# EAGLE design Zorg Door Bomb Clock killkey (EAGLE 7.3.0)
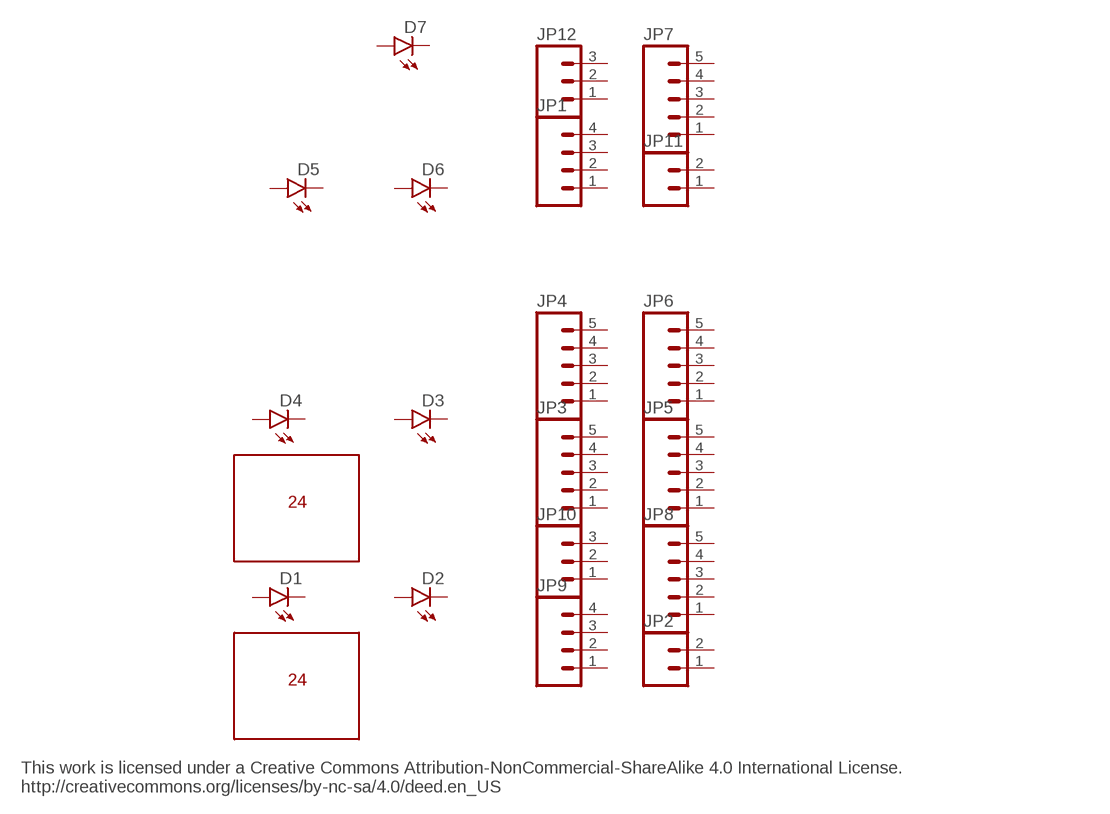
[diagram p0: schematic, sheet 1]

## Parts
D1  LED1206  [LED-1206]
D2  LED1206  [LED-1206]
D3  LED1206  [LED-1206]
D4  LED1206  [LED-1206]
D5  LED1206  [LED-1206]
D6  LED1206  [LED-1206]
D7  LED1206  [LED-1206]
JP1  M041X04_NO_SILK  [1X04_NO_SILK]
JP2  M021X02_NO_SILK  [1X02_NO_SILK]
JP3  M05NO_SILK  [1X05_NO_SILK]
JP4  M05NO_SILK  [1X05_NO_SILK]
JP5  M05NO_SILK  [1X05_NO_SILK]
JP6  M05NO_SILK  [1X05_NO_SILK]
JP7  M05NO_SILK  [1X05_NO_SILK]
JP8  M05NO_SILK  [1X05_NO_SILK]
JP9  M041X04_NO_SILK  [1X04_NO_SILK]
JP10  M031X03_NO_SILK  [1X03_NO_SILK]
JP11  M021X02_NO_SILK  [1X02_NO_SILK]
JP12  M031X03_NO_SILK  [1X03_NO_SILK]
U$1  SOIC24  [SOIC24]
U$2  SOIC24  [SOIC24]
Unconnected: D1.A D1.C D2.A D2.C D3.A D3.C D4.A D4.C D5.A D5.C D6.A D6.C D7.A D7.C JP1.1 JP1.2 JP1.3 JP1.4 JP2.1 JP2.2 JP3.1 JP3.2 JP3.3 JP3.4 JP3.5 JP4.1 JP4.2 JP4.3 JP4.4 JP4.5 JP5.1 JP5.2 JP5.3 JP5.4 JP5.5 JP6.1 JP6.2 JP6.3 JP6.4 JP6.5 JP7.1 JP7.2 JP7.3 JP7.4 JP7.5 JP8.1 JP8.2 JP8.3 JP8.4 JP8.5 JP9.1 JP9.2 JP9.3 JP9.4 JP10.1 JP10.2 JP10.3 JP11.1 JP11.2 JP12.1 JP12.2 JP12.3

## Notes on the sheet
- This work is licensed under a Creative Commons Attribution-NonCommercial-ShareAlike 4.0 International License.
  http://creativecommons.org/licenses/by-nc-sa/4.0/deed.en_US

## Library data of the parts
D1-D7 = SparkFun-LED:LED: LEDs
JP1 JP9 = zorg header 1:M04: Header 4 Standard 4-pin 0.1" header. Use with straight break away headers (SKU : PRT-00116), right angle break away headers (PRT-00553), swiss pins (PRT-00743), machine pins (PRT-00117), and female headers (PRT-00115). Molex polarized connector foot print use with SKU : PRT-08231 with associated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; PROD_ID: CONN-09696
JP2 JP11 = zorg header 1:M02: Standard 2-pin 0.1" header. Use with
JP3-JP8 = zorg header 1:M05: Header 5 Standard 5-pin 0.1" header. Use with straight break away headers (SKU : PRT-00116), right angle break away headers (PRT-00553), swiss pins (PRT-00743), machine pins (PRT-00117), and female headers (PRT-00115). Molex polarized connector foot print use with SKU : PRT-08230 with associated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
JP10 JP12 = zorg header 1:M03: Header 3 Standard 3-pin 0.1" header. Use with straight break away headers (SKU : PRT-00116), right angle break away headers (PRT-00553), swiss pins (PRT-00743), machine pins (PRT-00117), and female headers (PRT-00115). Molex polarized connector foot print use with SKU : PRT-08232 with associated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
U$1 U$2 = soic24:SOIC24

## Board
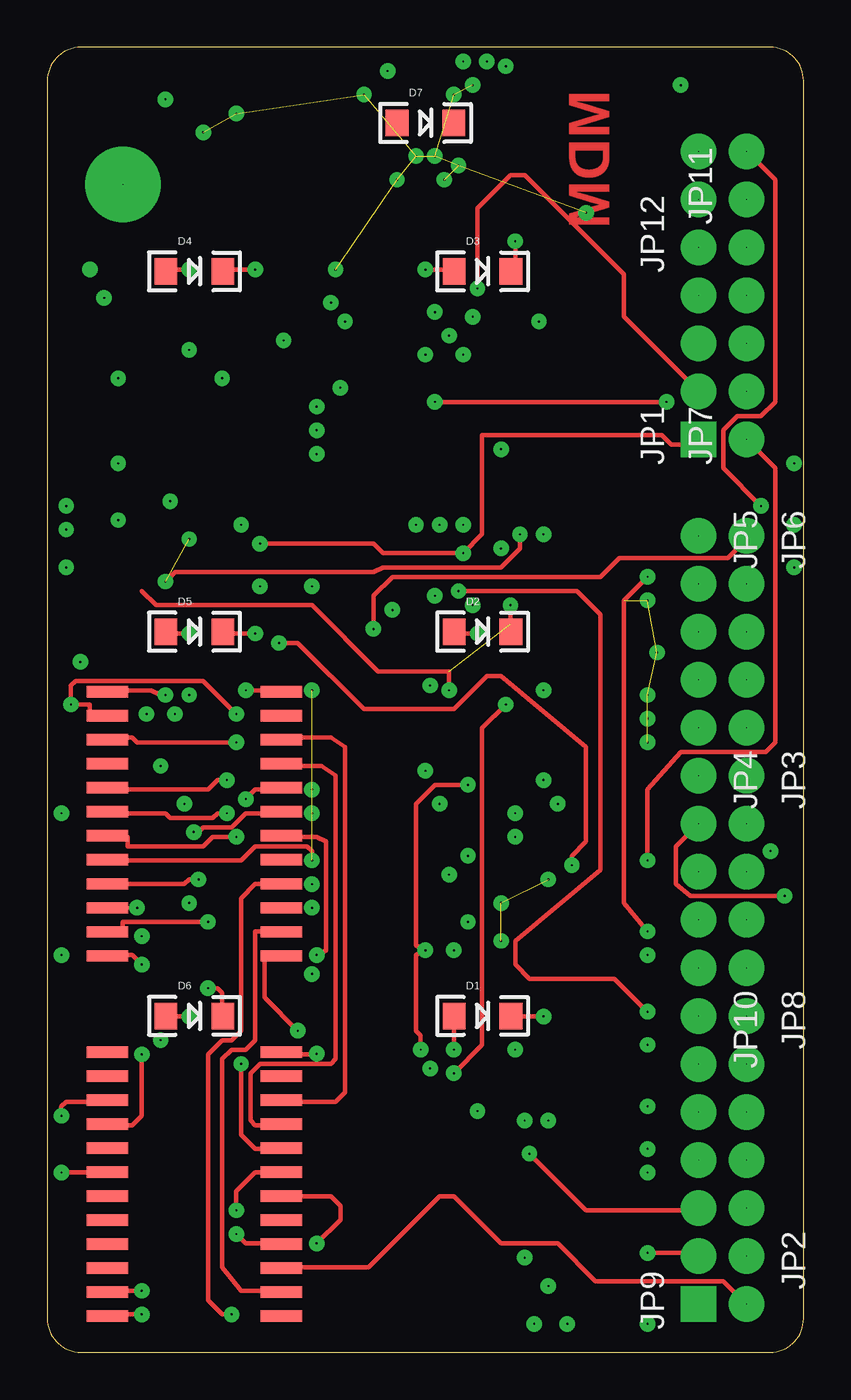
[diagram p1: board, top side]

Size 40 x 69 mm. Coordinates in mm from the lower left corner, seen from the top.
Outline: 0,67.23 0,1.77 arc90 1.77,0 38.23,0 arc90 40,1.77 40,67.23 arc90 38.23,69 1.77,69 arc90 0,67.23
Copper layers (1*16): Top 0.035mm / dielectric 1.5mm / Bottom 0.035mm
Design rules "default": minimum track width 10mil, minimum drill 24mil, track to track 8mil, track to pad 8mil, pad to pad 8mil, via to via 8mil, smd to smd 8mil, copper to edge 40mil, drill to drill 8mil, minimum pad ring 10mil, minimum via ring 8mil, stop-mask expansion 4mil, vias tented up to drill 0mil, thermal gap 10mil

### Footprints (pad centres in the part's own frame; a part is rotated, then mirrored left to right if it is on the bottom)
LED-1206 = smd 1.2 x 1.4: A -1.5,0; C 1.5,0
1X04_NO_SILK = drill 0.003 pad 1.88 square: 1 0,0 | drill 0.003 pad 1.88: 2 2.54,0; 3 5.08,0; 4 7.62,0
1X02_NO_SILK = drill 0.025 pad 1.88: 1 0,0; 2 2.54,0
1X05_NO_SILK = drill 0.025 pad 1.88: 1 0,0; 2 2.54,0; 3 5.08,0; 4 7.62,0; 5 10.16,0
1X03_NO_SILK = drill 0.025 pad 1.88: 1 0,0; 2 2.54,0; 3 5.08,0
SOIC24 = smd 2.2 x 0.6: 1 10.95,0.635; 2 10.95,1.905; 3 10.95,3.175; 4 10.95,4.445; 5 10.95,5.715; 6 10.95,6.985; 7 10.95,8.255; 8 10.95,9.525; 9 1.75,9.525; 10 1.75,8.255; 11 1.75,6.985; 12 1.75,5.715; 13 1.75,4.445; 14 1.75,3.175; 15 1.75,1.905; 16 1.75,0.635; 17 10.95,12.065; 18 1.75,14.605; 19 10.95,10.795; 20 10.95,13.335; 21 10.95,14.605; 22 1.75,13.335; 31 1.75,12.065; 32 1.75,10.795

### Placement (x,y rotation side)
D1  23.02,17.78 0 top
D2  23.02,38.1 0 top
D3  23.02,57.15 0 top
D4  7.78,57.15 0 top
D5  7.78,38.1 0 top
D6  7.78,17.78 0 top
D7  20,65 0 top
JP1  34.45,48.26 90 top
JP2  36.99,5.08 270 top
JP3  36.99,30.48 270 top
JP4  34.45,30.48 270 top
JP5  34.45,43.18 270 top
JP6  36.99,43.18 270 top
JP7  36.99,48.26 90 top
JP8  36.99,17.78 270 top
JP9  34.45,2.54 90 top
JP10  34.45,17.78 270 top
JP11  36.99,60.96 90 top
JP12  34.45,58.42 90 top
U$1  1.43,20.32 0 top
U$2  1.43,1.27 0 top

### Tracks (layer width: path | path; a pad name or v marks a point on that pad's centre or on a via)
N$1  (via drill 0.1 pad 0.81)
  Top 0.229: 2.25,33.75 2.25,34.25 v1.25,34.25 1.25,35.25 1.5,35.5 8.25,35.5 v10,33.75
N$2  (via drill 0.1 pad 0.81)
  other vias: 5.25,33.75
N$3  (via drill 0.1 pad 0.81)
  other vias: 6.25,34.75
N$4  (via drill 0.1 pad 0.81)
  other vias: 6.75,33.75
N$5  (via drill 0.1 pad 0.81)
  other vias: 7.5,34.75
N$6
  Top 0.229: 3.25,35 5.5,35 6,34.75
N$7  (via drill 0.1 pad 0.81)
  Top 0.229: v10.5,35 12.25,35
N$8  (via drill 0.1 pad 0.81)
  other vias: 10,32.25
N$9  (via drill 0.1 pad 0.81)
  other vias: 6,31
N$10  (via drill 0.1 pad 0.81)
  Top 0.229: 12.25,29.75 11,29.75 v10.5,29.25
N$11  (via drill 0.1 pad 0.81)
  other vias: 9.5,30.25
N$12
  Top 0.229: 4,26 10.25,26 11,26.75 13.75,26.75 14,26.5 14,26
N$13  (via drill 0.1 pad 0.81)
  other vias: 7.25,29
N$14  (via drill 0.1 pad 0.81)
  Top 0.229: v7.75,27.5 8,27.5 8.25,27.75 9.75,27.75 10.5,28.5 12,28.5
N$15  (via drill 0.1 pad 0.81)
  other vias: 10,27.25
N$16  (via drill 0.1 pad 0.81)
  other vias: 0.75,28.5
N$17  (via drill 0.1 pad 0.81)
  other vias: 0.75,21
N$18  (via drill 0.1 pad 0.81)
  other vias: 5,20.5
N$19  (via drill 0.1 pad 0.81)
  other vias: 5,22
N$20  (via drill 0.1 pad 0.81)
  Top 0.178: 3.75,23.5 v4.75,23.5
N$21  (via drill 0.1 pad 0.81)
  other vias: 7.5,23.75
N$22  (via drill 0.1 pad 0.81)
  other vias: 8.5,22.75
N$23
  Top 0.229: 3.75,32.5 4.5,32.5 4.75,32.25 10,32.25
N$24
  Top 0.229: 4,29.75 8.5,29.75 9,30.25 9.5,30.25
N$25  (via drill 0.1 pad 0.81)
  Top 0.229: 3.75,28.5 6.25,28.5 6.5,28.25 8.75,28.25 9,28.5 v9.5,28.5
N$26
  Top 0.229: 4.25,27.25 4.25,26.75 8.25,26.75 8.75,27.25 10,27.25
N$27  (via drill 0.1 pad 0.81)  (1 unrouted)
  other vias: 14,35 14,26
N$28
  Top 0.229: 37,2.5 35.75,3.75 29,3.75 27,5.75 24,5.75 21.5,8.25 20.75,8.25 17,4.5 12.5,4.5
N$29
  Top 0.229: 12.25,32.5 15,32.5 15.75,32 15.75,13.75 15.25,13.25 12.5,13.25
N$30  (via drill 0.1 pad 0.81)
  other vias: 14,29.75
N$31  (via drill 0.1 pad 0.81)
  other vias: 14,28.5
N$32  (via drill 0.1 pad 0.81)
  other vias: 14,24.75
N$33  (via drill 0.1 pad 0.81)
  other vias: 14,23.5
N$34  (via drill 0.1 pad 0.81)
  other vias: 14,20
N$35
  Top 0.229: 4,22.5 4,22.75 8.5,22.75
N$36  (via drill 0.1 pad 0.81)
  Top 0.229: 13,27.25 14.25,27.25 14.75,27 14.75,21.25 v14.25,21
N$37
  Top 0.229: 3.75,21 4.5,21 5,20.5
N$38  (via drill 0.1 pad 0.81)
  Top 0.229: 3.5,24.75 7.25,24.75 7.5,25 v8,25
N$39  (via drill 0.1 pad 0.81)
  Top 0.229: 9.25,18 9.25,19 9,19.25 v8.5,19.25
N$40  (via drill 0.1 pad 0.81)
  Top 0.229: 6.25,17.75 v7.5,17.75
N$41
  Top 0.229: 12.75,15.75 14.25,15.75
N$42  (via drill 0.1 pad 0.81)
  other vias: 6,16.5
N$43  (via drill 0.1 pad 0.81)
  other vias: 0.75,12.5
N$44
  Top 0.229: 0.75,12.75 0.75,13 1,13.25 3.25,13.25
N$45  (via drill 0.1 pad 0.81)
  Top 0.229: 3.25,12 4.5,12 5,12.5 v5,15.75
N$46  (via drill 0.1 pad 0.81)
  Top 0.229: 11.5,21 11.5,18.75 v13.25,17
N$47  (via drill 0.1 pad 0.81)
  other vias: 14.25,15.78
N$48
  Top 0.229: 11.5,22.25 11,22.25 11,16.5 10.5,16 9.75,16 9.25,15.5 9.25,4.5 10.25,3.25 12.25,3.25 | 3,3.25 5,3.25 | 3,2 5,2
N$49  (via drill 0.1 pad 0.81)
  Top 0.229: v10.25,15.25 10.25,11.5 11,10.75 12,10.75
N$50  (via drill 0.1 pad 0.81)
  Top 0.229: 12,24.75 11,24.75 10.25,24 10.25,17 9.75,16.5 9.25,16.5 8.5,15.75 8.5,2.75 9.25,2 v9.75,2
N$51
  Top 0.229: 11.75,12 11,12 10.75,12.25 10.75,14.75 11.25,15.25 15,15.25 15.25,15.5 15.25,30.5 14.5,31 12.5,31
N$52  (via drill 0.1 pad 0.81)
  Top 0.229: v0.75,9.5 1.5,9.5 2.75,9.5
N$53  (via drill 0.1 pad 0.81)
  Top 0.229: 34.5,5.25 v31.75,5.25
N$54  (via drill 0.1 pad 0.81)
  Top 0.229: v14.25,5.75 15.5,7 15.5,7.75 15,8.25 12.25,8.25
N$55  (via drill 0.1 pad 0.81)
  Top 0.229: 12.25,5.75 10.5,5.75 v10,6.25
N$56  (via drill 0.1 pad 0.81)
  Top 0.229: 11.75,9.5 11,9.5 10,8.5 v10,7.5
N$57  (via drill 0.1 pad 0.81)
  Top 0.229: 34.5,7.5 28.5,7.5 v25.5,10.5
N$58  (via drill 0.1 pad 0.81)
  other vias: 25.25,5
N$59  (via drill 0.1 pad 0.81)
  other vias: 26.5,3.5
N$60  (via drill 0.1 pad 0.81)
  other vias: 25.75,1.5
N$61  (via drill 0.1 pad 0.81)
  other vias: 27.5,1.5
N$62  (via drill 0.1 pad 0.81)
  other vias: 31.75,1.5
N$63  (via drill 0.1 pad 0.81)
  other vias: 31.75,9.5
N$64  (via drill 0.1 pad 0.81)
  other vias: 31.75,10.75
N$65  (via drill 0.1 pad 0.81)
  other vias: 31.75,13
N$66  (via drill 0.1 pad 0.81)
  other vias: 31.75,16.25
N$67  (via drill 0.1 pad 0.81)
  other vias: 25.25,12.25
N$68  (via drill 0.1 pad 0.81)
  other vias: 26.5,12.25
N$69  (via drill 0.1 pad 0.81)
  Top 0.229: v21.5,16 21.5,17.5
N$70  (via drill 0.1 pad 0.81)
  other vias: 24.75,16
N$71  (via drill 0.1 pad 0.81)
  Top 0.229: v26.25,17.75 24.75,17.75
N$72  (via drill 0.1 pad 0.81)
  Top 0.229: v21.5,14.75 23,16.25 23,33 v24.25,34.25
N$73  (via drill 0.1 pad 0.81)
  other vias: 20.25,15
N$74
  Top 0.229: 34.5,50.75 30.5,54.75 30.5,57 25.25,62.25 24.5,62.25 22.75,60.5 22.75,56
N$75  (via drill 0.1 pad 0.81)
  Top 0.229: v31.75,18 30,19.75 25.5,19.75 24.75,20.5 24.75,21.75 29.25,25.5 29.25,39 28,40.25 v21.75,40.25
N$76  (via drill 0.1 pad 0.81)
  other vias: 31.75,21
N$77  (via drill 0.1 pad 0.81)
  other vias: 31.75,22.25
N$78  (via drill 0.1 pad 0.81)
  Top 0.229: v39,24.13 34,24.13 33.25,24.75 33.25,26.75 34.5,28
N$79  (via drill 0.1 pad 0.81)
  other vias: 38.25,26.5
N$80  (via drill 0.1 pad 0.81)
  Top 0.229: v31.75,26 31.75,29.75 33.5,31.75 38,31.75 38.5,32.25 38.5,46.75 37,48.25
N$81  (via drill 0.1 pad 0.81)
  Top 0.178: 37,43.25 37,43
  Top 0.229: 37,43 36,42 30.25,42 29.25,41 18.25,41 17.25,40 v17.25,38.25
N$82  (via drill 0.1 pad 0.81)
  Top 0.229: v7.5,38 6.25,38
N$83  (via drill 0.1 pad 0.81)
  Top 0.229: v11,38 9.5,38
N$84  (via drill 0.1 pad 0.81)
  Top 0.229: v12.25,37.5 13.25,37.5 16.75,34 21.5,34 23.25,35.75 24,35.75 28.5,32 28.5,27 27.75,26.25 v27.75,25.75
N$85  (via drill 0.1 pad 0.81)  (2 unrouted)
  other vias: 26.5,25 24,23.75 24,21.75
N$86  (via drill 0.1 pad 0.81)
  other vias: 24.75,27.25
N$87  (via drill 0.1 pad 0.81)
  other vias: 24.75,28.5
N$88  (via drill 0.1 pad 0.81)
  other vias: 27,29
N$89  (via drill 0.1 pad 0.81)
  other vias: 26.25,30.25
N$90  (via drill 0.1 pad 0.81)
  other vias: 26.25,35
N$91  (via drill 0.1 pad 0.81)
  Top 0.229: v22.75,38 21.25,38
N$92  (via drill 0.1 pad 0.81)
  other vias: 22.5,39.5
N$93  (via drill 0.1 pad 0.81)
  other vias: 24.5,39.5
N$94  (via drill 0.1 pad 0.81)
  Top 0.229: 24.75,57.75 v24.75,58.75
N$95  (via drill 0.1 pad 0.81)
  other vias: 20.5,40
N$96  (via drill 0.1 pad 0.81)
  other vias: 18.25,39.25
N$97  (via drill 0.1 pad 0.81)  (1 unrouted)
  Top 0.229: 5,40.25 5.75,39.5 14,39.5 17.5,36 21.25,36 v21.25,35 | 24.5,39.5 24.5,38.5
N$98  (via drill 0.1 pad 0.81)
  other vias: 20.25,35.25
N$99  (via drill 0.1 pad 0.81)  (5 unrouted)
  Top 0.229: v31.75,41 30.5,39.75 30.5,23.75 31.75,22.25
  other vias: 31.75,39.75 32.25,37 31.75,32.25 31.75,33.5 31.75,34.75
N$100  (via drill 0.1 pad 0.81)
  Top 0.229: v22.25,30 20.5,30 19.5,29 19.5,21.5 v20,21.25 19.5,21 19.5,17 19.75,16.75 v19.75,16
N$101  (via drill 0.1 pad 0.81)
  other vias: 21.5,21.25
N$102  (via drill 0.1 pad 0.81)
  other vias: 22.25,22.75
N$103  (via drill 0.1 pad 0.81)
  other vias: 21.25,25.25
N$104  (via drill 0.1 pad 0.81)
  other vias: 22.25,26.25
N$105  (via drill 0.1 pad 0.81)
  other vias: 20.75,29
N$106  (via drill 0.1 pad 0.81)
  other vias: 20,30.75
N$107  (via drill 0.1 pad 0.81)
  other vias: 22.75,12.75 5,2 5,3.25
N$108  (via drill 0.1 pad 0.81)
  other vias: 1.75,36.5
N$109  (via drill 0.1 pad 0.81)
  other vias: 1,41.5
N$110  (via drill 0.1 pad 0.81)
  other vias: 1,43.5
N$111  (via drill 0.1 pad 0.81)
  other vias: 1,44.75
N$112  (via drill 0.1 pad 0.81)
  other vias: 3.75,44
N$113  (via drill 0.1 pad 0.81)
  Top 0.229: 6.25,40.75 6.75,41.25 17.25,41.25 17.75,41.5 24,41.5 25,42.5 v25,43.25
N$114  (via drill 0.1 pad 0.81)
  other vias: 24,42.5
N$115  (via drill 0.1 pad 0.81)
  other vias: 26.25,43.25
N$116  (via drill 0.1 pad 0.81)
  other vias: 11.25,40.5
N$117  (via drill 0.1 pad 0.81)
  other vias: 14,40.5
N$118  (via drill 0.1 pad 0.81)
  other vias: 22.75,56.25
N$119  (via drill 0.1 pad 0.81)
  other vias: 22,43.75
N$120  (via drill 0.1 pad 0.81)
  other vias: 20.75,43.75
N$121  (via drill 0.1 pad 0.81)
  other vias: 19.5,43.75
N$122  (via drill 0.1 pad 0.81)
  Top 0.229: 34.5,48 33,48 32.5,48.5 23,48.5 23,43.25 v22,42.25 17.75,42.25 17.25,42.75 v11.25,42.75
N$123  (via drill 0.1 pad 0.81)
  other vias: 24,47.75
N$124  (via drill 0.1 pad 0.81)
  other vias: 10.25,43.75
N$125  (via drill 0.1 pad 0.81)  (1 unrouted)
  other vias: 7.5,43 6.25,40.75
N$126  (via drill 0.1 pad 0.81)
  other vias: 6.5,45
N$127  (via drill 0.1 pad 0.81)
  other vias: 3.75,47
N$128  (via drill 0.1 pad 0.81)
  other vias: 14.25,48.75
N$129  (via drill 0.1 pad 0.81)
  other vias: 14.25,50
N$130  (via drill 0.1 pad 0.81)
  Top 0.229: v32.75,50.25 v20.5,50.25
N$131  (via drill 0.1 pad 0.81)
  Top 0.229: v20,57.25 21.5,57.25
N$132  (via drill 0.1 pad 0.81)
  other vias: 26,54.5
N$133  (via drill 0.1 pad 0.81)
  other vias: 22.5,54.75
N$134  (via drill 0.1 pad 0.81)
  other vias: 20.5,55
N$135  (via drill 0.1 pad 0.81)
  other vias: 21.25,53.75
N$136  (via drill 0.1 pad 0.81)
  other vias: 22,52.75
N$137  (via drill 0.1 pad 0.81)
  other vias: 20,52.75
N$138  (via drill 0.1 pad 0.81)  (11 unrouted)
  other vias: 15.25,57.25 19.5,63.25 20.5,63.25 21.75,62.75 21,62 18.5,62 8.25,64.5 10,65.5 16.75,66.5 21.5,66.5 22.5,67 28.5,60.25
N$139  (via drill 0.1 pad 0.81)
  other vias: 15,55.5
N$140  (via drill 0.1 pad 0.81)
  other vias: 15.75,54.5
N$141  (via drill 0.1 pad 0.81)
  other vias: 12.5,53.5
N$142  (via drill 0.1 pad 0.81)
  other vias: 15.5,51
N$143  (via drill 0.1 pad 0.81)
  other vias: 14.25,47.5
N$144  (via drill 0.1 pad 0.81)
  other vias: 7.5,53
N$145  (via drill 0.1 pad 0.81)
  Top 0.229: v7.5,57.25 6.25,57.25
N$146  (via drill 0.1 pad 0.81)
  other vias: 9.25,51.5
N$147  (via drill 0.1 pad 0.81)
  other vias: 3.75,51.5
N$148  (via drill 0.1 pad 0.81)
  Top 0.229: v11,57.25 9.25,57.25
N$149  (via drill 0.1 pad 0.81)
  other vias: 3,55.75
N$150  (via drill 0.01 pad 0.81)
  other vias: 2.25,57.25
N$151  (via drill 0.01 pad 4)
  other vias: 4,61.75
N$152  (via drill 0.1 pad 0.81)
  Top 0.229: v37.75,44.75 35.75,46.75 35.75,48.75 36.5,49.5 37.75,49.5 38.5,50.25 38.5,62 37,63.5
N$153  (via drill 0.1 pad 0.81)
  other vias: 39.5,47
N$154  (via drill 0.1 pad 0.81)
  other vias: 39.5,43.75
N$155  (via drill 0.1 pad 0.81)
  other vias: 39.5,41.5
N$156  (via drill 0.1 pad 0.81)
  other vias: 6.25,66.25
N$157  (via drill 0.1 pad 0.81)
  other vias: 18,67.75
N$158  (via drill 0.1 pad 0.81)
  other vias: 22,68.25
N$159  (via drill 0.1 pad 0.81)
  other vias: 23.25,68.25
N$160  (via drill 0.1 pad 0.81)
  other vias: 24.25,68
N$161  (via drill 0.1 pad 0.81)
  other vias: 33.5,67

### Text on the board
Top: MDM
Unrouted: This work is licensed under a Creative Commons Attribution-NonCommercial-ShareAlike 4.0 International License. / http://creativecommons.org/licenses/by-nc-sa/4.0/deed.en_US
